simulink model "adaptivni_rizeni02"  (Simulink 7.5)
settings: Solver=ode45  StartTime=0.0  StopTime=100  RelTol=1e-3

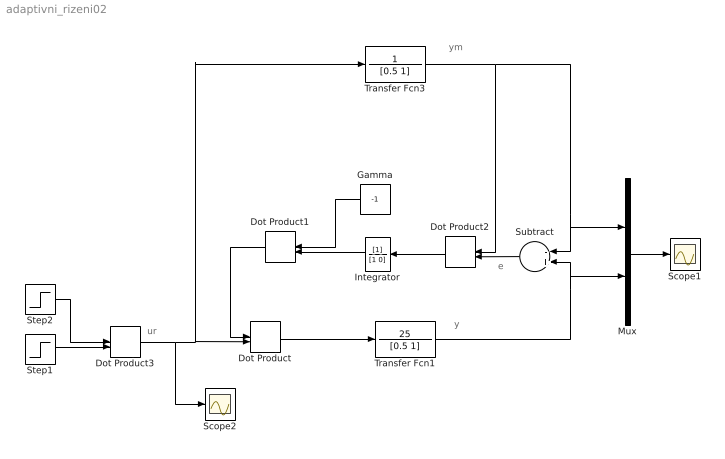
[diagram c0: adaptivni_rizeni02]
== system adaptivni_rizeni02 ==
  note: ur
  note: e
  note: ym
  note: y
  Dot Product{,1..3} (4 alike) : DotProduct  OutDataType=sfix(16)  OutScaling=2^-10
  Gamma : Constant  Value=-1  OutDataType=sfix(16)  OutScaling=2^0
  Integrator : TransferFcn  Denominator=[1 0]
  Mux : Mux  Inputs=2
  Scope1 : Scope
  Scope2 : Scope
  Step1 : Step  Time=0  SampleTime=0
  Step2 : Step  Time=25  Before=1  After=2  SampleTime=0
  Subtract : Sum  Inputs=-+  OutDataType=sfix(16)  OutScaling=2^-10
  Transfer Fcn1 : TransferFcn  Numerator=25  Denominator=[0.5 1]
  Transfer Fcn3 : TransferFcn  Numerator=1  Denominator=[0.5 1]
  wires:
  Integrator/1 -> Dot Product1/2
  Gamma/1 -> Dot Product1/1
  Dot Product2/1 -> Integrator/1
  Subtract/1 -> Dot Product2/2
  Dot Product1/1 -> Dot Product/1
  Dot Product/1 -> Transfer Fcn1/1
  Dot Product3/1 -> Dot Product/2, Transfer Fcn3/1, Scope2/1
  Transfer Fcn3/1 -> Dot Product2/1, Subtract/1, Mux/1
  Mux/1 -> Scope1/1
  Step1/1 -> Dot Product3/2
  Step2/1 -> Dot Product3/1
  Transfer Fcn1/1 -> Subtract/2, Mux/2
